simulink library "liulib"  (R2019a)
settings: Solver=ode45  StartTime=0.0  StopTime=10.0  RelTol=1e-3  EnableMultiTasking=on
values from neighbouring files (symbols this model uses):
  ag = ones(ng,1); [fPg,fTg] = bfgenD(0,P)    [bfgenD.m]    (also in fbtfit.m = AA \ [Ip ; rBt^2 ; 0]; fbtt.m = zeros(L.ng,1); fgeFpicard.m = x(2+(1:L.ng)))
  aq = []    [fbtt.m]
  aW = []    [fbtt.m]
  D = Fyi1j + Fyim1j + A.*Fyij1  +B.*Fyijm1 - C.*Fyij    [dlst.m]    (also in fbtp.m = meqp(); fgep.m = fgsp(P,varargin{:}))
  dr2FA = dr2Fs(1:nA,1)    [asxycs.m]
  drzFA = drzFs(1:nA,1)    [asxycs.m]
  dz = (z - zx(kz))/dzx    [bintc.m]
  dz2FA = dz2Fs(1:nA,1)    [asxycs.m]
  FA = Fs(1:nA,1)    [asxycs.m]    (also in bfhelp.m = [-1                        0      	 0])
  FB = [0                         1        1]    [bfhelp.m]
  Fx = zeros(n+2,3); Fx(2:end-1,2) = FN    [bfhelp.m]    (also in fbtt.m = meqFx(L,Iy,[Ia;Iu]); fgeFpicard.m = FxP + Fxe)
  FX = Fs(nA+1:ns,1)    [asxycs.m]
  Ie = [Ia;Iu]    [fgeF.m]    (also in fgeFpicard.m = (L.Mee + diag(LXt.dt*L.Re))\       ([LXt.dt*LXt.Va;zeros(L.G)
  IpD = LX.IpD(:,kt)    [fbtt.m]    (also in fgeFpicard.m = LXt.(L.agconc{1,3}))
  Iy = (Iy+flipud(Iy))*0.5    [fbtt.m]    (also in fgeF.m = reshape( xnl(L.ind.iy) , L.nzy, L.nry); fgeFpicard.m = Iyscal*reshape(Tyg*ag,L.nzy,L.nry))
  L = fbtc(P,G)    [fbt.m]    (also in fbtc.m = meqc(P,G,'rrx','zzx'); fbte.m = varargout{1}; fge.m = fgel(L,meqxk(LX,1)); fgec.m = fgsc(P,G))
  lB = false    [fbtt.m]
  lX = false    [fbtt.m]
  nA = numel(rA)    [asxycs.m]    (also in fbtt.m; fgeFpicard.m)
  niter = L.P.itercs    [asxycs.m]    (also in fbtt.m = 2)
  Opy = zeros(meqsize(L, 'Opy'),'int8')    [fbtt.m]
  rA = rs(1:nA,1)    [asxycs.m]    (also in fbtptcv.m = (rA1 + 3*rA2)/4)
  rBt = LX.rBt(kt)    [fbtt.m]    (also in fgeFpicard.m = LXt.rBt)
  rX = rs(nA+1:ns,1)    [asxycs.m]    (also in fbtptcv.m = rzbro(iX,1); fbtxana.m = r0 + [1; 1]*a0*0.5)
  zA = zs(1:nA,1)    [asxycs.m]    (also in fbtptcv.m = (zA1 + 3*zA2)/4)
  zX = zs(nA+1:ns,1)    [asxycs.m]    (also in fbtptcv.m = rzbro(iX,2); fbtxana.m = z0 + [1;-1]*a0*1.0)
undefined symbols (not defined in the file or in its folder): aminor, Bm, bp, bpli2, Brn, Brrn, Brzn, bt, Bzn, Bzrn, Bzzn, delta, deltal, deltau, dzg, epsilon, err, Ff, Fn, Ft, Ft0, FW, Ip, iqQ, iTQ, jtorQ, kappa, li, lp, mu, nX, PpQ, PQ, Q0Q, Q1Q, Q2Q, Q3Q, Q4Q, q95, qmin, raQ, raqmin, rB, rbary, repmat, rgeom, rIp, rIpD, Row, rq, rS, rst, TQ, TTpQ, vector, Vn, Vp, Wk, WN, Wp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
libraries: $bdroot x52, mkllib x48, simulink x7
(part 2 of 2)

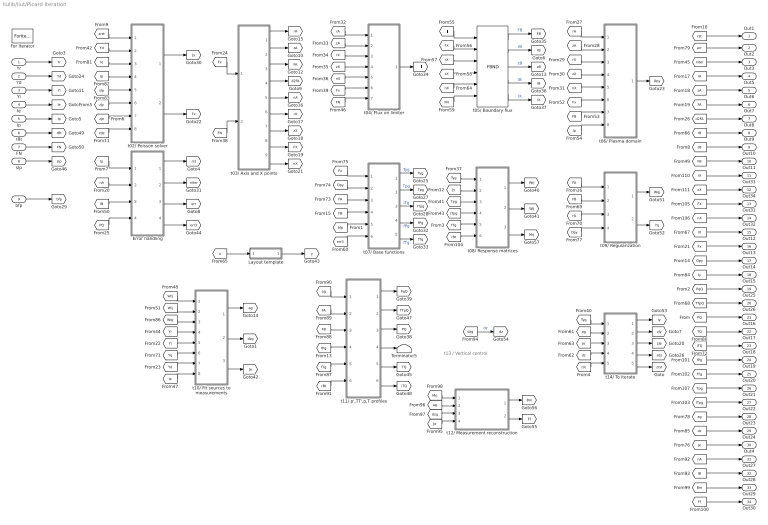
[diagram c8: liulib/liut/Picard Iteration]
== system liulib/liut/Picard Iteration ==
  note: t13 / Vertical control
  Yr : Inport
  Yd : Inport  Port=2
  Yi : Inport  Port=3
  Ie : Inport  Port=4
  Ip : Inport  Port=5
  rBt : Inport  Port=6
  FN : Inport  Port=7
  sIp : Inport  Port=8
  bfp : Inport  Port=9
  Error handling : Subsystem
  For Iterator : ForIterator  IterationLimit=L.P.itert  ShowIterationPort=off
  Layout template : Subsystem  Commented=on
  Terminator5 : Terminator
  t02/ Poisson solver : Subsystem
  t03/ Axis and X points : Subsystem  TreatAsAtomicUnit=on
  t04/ Flux on limiter : Subsystem
  t05/ Boundary flux : $bdroot/FBND  rl=L.G.rl  zl=L.G.zl
  t06/ Plasma domain : Subsystem
  t07/ Base functions : Subsystem  Variant=on
  t08/ Response matrices : Subsystem
  t09/ Regularization : Subsystem  TreatAsAtomicUnit=on
  t10/ Fit sources to measurements : Subsystem  Variant=on  VariantControl=Variant1
  t11/ p',TT',p,T profiles : Subsystem  VariantControl=Variant1
  t12/ Measurement reconstruction : Subsystem
  t14/ To iterate : Subsystem
  Out1 : Outport
  Out2 : Outport  Port=2
  Out3 : Outport  Port=3
  Out5 : Outport  Port=4
  Out6 : Outport  Port=5
  Out7 : Outport  Port=6
  Out8 : Outport  Port=7
  Out9 : Outport  Port=8
  Out10 : Outport  Port=9
  Out11 : Outport  Port=10
  Out33 : Outport  Port=11
  Out34 : Outport  Port=12
  Out31 : Outport  Port=13
  Out32 : Outport  Port=14
  Out12 : Outport  Port=15
  Out13 : Outport  Port=16
  Out14 : Outport  Port=17
  Out15 : Outport  Port=18
  Out25 : Outport  Port=19
  Out26 : Outport  Port=20
  Out16 : Outport  Port=21
  Out17 : Outport  Port=22
  Out18 : Outport  Port=23
  Out19 : Outport  Port=24
  Out20 : Outport  Port=25
  Out21 : Outport  Port=26
  Out22 : Outport  Port=27
  Out23 : Outport  Port=28
  Out24 : Outport  Port=29
  Out4 : Outport  Port=30
  Out27 : Outport  Port=31
  Out28 : Outport  Port=32
  Out29 : Outport  Port=33
  Out30 : Outport  Port=34
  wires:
  t03/ Axis and X points/9(nX) -> [nX]
  t03/ Axis and X points/8(FX) -> [FX]
  t03/ Axis and X points/7(zX) -> [zX]
  t03/ Axis and X points/6(rX) -> [rX]
  t03/ Axis and X points/5(nA) -> [nA]
  t03/ Axis and X points/4(d2FA) -> [d2FA]
  t03/ Axis and X points/3(FA) -> [FA]
  t03/ Axis and X points/2(zA) -> [zA]
  t03/ Axis and X points/1(rA) -> [rA]
  [FN] -> t03/ Axis and X points/2(FN)
  [Fx] -> t03/ Axis and X points/1(Fx)
  [zX] -> Out34/1
  [rX] -> Out33/1
  [nX] -> Out32/1
  [Bm] -> Out29/1
  [Ff] -> Out30/1
  [Je] -> t12/ Measurement reconstruction/4(Ie)
  t08/ Response matrices/3(Mrj) -> [Mrj]
  [dzg] -> t12/ Measurement reconstruction/3(dzg)
  [ag] -> t12/ Measurement reconstruction/2(ag)
  [Mrj] -> t12/ Measurement reconstruction/1(Mrj)
  t12/ Measurement reconstruction/2(Ff) -> [Ff]
  t12/ Measurement reconstruction/1(Bm) -> [Bm]
  [dzg] -> [dz]  "dz"
  [lB] -> Out28/1
  [nA] -> Out27/1
  t14/ To iterate/1(Iy) -> [Iy]
  [TTpQ] -> Out26/1
  [PqQ] -> Out25/1
  t14/ To iterate/5(zrst) -> [zrst]
  t14/ To iterate/4(zdz) -> [zdz]
  t14/ To iterate/3(zJe) -> [zJe]
  t14/ To iterate/2(zJy) -> [zJy]
  [dz] -> t14/ To iterate/4(dz)
  [Je] -> t14/ To iterate/3(Je)
  [Tyg] -> t14/ To iterate/1(Tyg)
  [ag] -> t14/ To iterate/2(ag)
  [rst] -> t14/ To iterate/5(rst)
  [fPg] -> t11/ p',TT',p,T profiles/4(fPg)
  [ag] -> t11/ p',TT',p,T profiles/1(ag)
  [FA] -> t11/ p',TT',p,T profiles/2(FA)
  [ITpg] -> Out22/1
  rBt/1 -> [rBt]
  FN/1 -> [FN]
  [zB] -> Out10/1
  Error handling/2(niter) -> [niter]
  Error handling/1(rst) -> [rst]
  t08/ Response matrices/1(Wrj) -> [Wrj]
  [Fx] -> t07/ Base functions/1(Fx)
  [Opy] -> t07/ Base functions/2(Opy)
  [FA] -> t07/ Base functions/3(FA)
  t02/ Poisson solver/1(Jy) -> [Jy]
  [zdz] -> t02/ Poisson solver/8(zdz)
  t02/ Poisson solver/2(Fx) -> [Fx]
  [dz] -> Out24/1
  [niter] -> Out3/1
  [lB] -> Error handling/3(lB)
  Error handling/3(err) -> [err]
  [Fx] -> t06/ Plasma domain/6(Fx)
  [FB] -> t06/ Plasma domain/7(FB)
  [Ip] -> t06/ Plasma domain/8(Ip)
  [TQ] -> Out17/1
  [Ie] -> t02/ Poisson solver/3(Ie)
  [Ip] -> t02/ Poisson solver/4(Ip)
  [rBt] -> t11/ p',TT',p,T profiles/6(rBt)
  [err] -> Out2/1
  [ag] -> Out23/1
  [d2FA] -> Out8/1
  [FA] -> Out7/1
  [FB] -> t07/ Base functions/4(FB)
  [err3] -> t07/ Base functions/6(err)
  t07/ Base functions/1(Tyg) -> [Tyg]  "Tyg"
  [bfp] -> t07/ Base functions/5(bfp)
  t07/ Base functions/4(fPg) -> [fPg]  "fPg"
  t07/ Base functions/5(fTg) -> [fTg]  "fTg"
  t05/ Boundary flux/1 -> [FB]  "FB"
  t05/ Boundary flux/2 -> [rB]  "rB"
  t05/ Boundary flux/3 -> [zB]  "zB"
  t05/ Boundary flux/4 -> [lB]  "lB"
  sIp/1 -> [sIp]
  [sIp] -> t02/ Poisson solver/5(sIp)
  [rst] -> Out1/1
  [Jy] -> t08/ Response matrices/2(Jy)
  t06/ Plasma domain/1(Opy) -> [Opy]
  [Tyg] -> t08/ Response matrices/1(Tyg)
  [Tpg] -> t08/ Response matrices/3(Tpg)
  t11/ p',TT',p,T profiles/1(PpQ) -> [PqQ]
  t11/ p',TT',p,T profiles/2(TTpQ) -> [TTpQ]
  t11/ p',TT',p,T profiles/4(hqTQ) -> Terminator5/1
  [fTg] -> t08/ Response matrices/5(fTg)
  t08/ Response matrices/2(Wij) -> [Wij]
  [zA] -> t06/ Plasma domain/2(zA)
  [zX] -> t06/ Plasma domain/4(zX)
  [nX] -> t06/ Plasma domain/5(nX)
  t11/ p',TT',p,T profiles/5(TQ) -> [TQ]
  t11/ p',TT',p,T profiles/6(iTQ) -> [iTQ]
  [iTQ] -> Out18/1
  [zJy] -> t02/ Poisson solver/6(zJy)
  [Yd] -> t02/ Poisson solver/2(Yd)
  [zJe] -> t02/ Poisson solver/7(zJe)
  Yr/1 -> [Yr]
  Yi/1 -> [Yi]
  Ip/1 -> [Ip]
  bfp/1 -> [bfp]
  [FN] -> t04/ Flux on limiter/7(FN)
  [Fx] -> t04/ Flux on limiter/6(Fx)
  [Fl] -> t05/ Boundary flux/1
  Yd/1 -> [Yd]
  Ie/1 -> [Ie]
  [zrst] -> t02/ Poisson solver/1(rst)
  [FB] -> t11/ p',TT',p,T profiles/3(FB)
  [fTg] -> t11/ p',TT',p,T profiles/5(fTg)
  t05/ Boundary flux/5 -> [lX]  "lX"
  [rA] -> t06/ Plasma domain/1(rA)
  [rX] -> t06/ Plasma domain/3(rX)
  [zX] -> t04/ Flux on limiter/4(zX)
  [rX] -> t04/ Flux on limiter/3(rX)
  [nX] -> t04/ Flux on limiter/5(nX)
  [Tpg] -> Out21/1
  [fTg] -> Out20/1
  [fPg] -> Out19/1
  [ITpg] -> t08/ Response matrices/4(ITpg)
  t04/ Flux on limiter/1(Fl) -> [Fl]
  [zA] -> Out6/1
  [rA] -> Out5/1
  [nX] -> t05/ Boundary flux/5
  [rB] -> Out9/1
  [lX] -> Out12/1
  t11/ p',TT',p,T profiles/3(PQ) -> [PQ]
  [Opy] -> Out14/1
  [FB] -> Out11/1
  [Fx] -> Out13/1
  [Ip] -> Error handling/1(Ip)
  [nA] -> Error handling/2(nA)
  [PQ] -> Error handling/4(PQ)
  [Iy] -> Out15/1
  [PQ] -> Out16/1
  [rX] -> t05/ Boundary flux/3
  [FX] -> t05/ Boundary flux/2
  [zX] -> t05/ Boundary flux/4
  Layout template/1(y) -> [y]
  [u] -> Layout template/1(u)
  [FN] -> t05/ Boundary flux/6
  [rA] -> t04/ Flux on limiter/1(rA)
  [zA] -> t04/ Flux on limiter/2(zA)
  t07/ Base functions/2(Tpg) -> [Tpg]  "Tpg"
  t07/ Base functions/3(ITpg) -> [ITpg]  "iTg"
  Error handling/4(err3) -> [err3]
  [Wrj] -> t10/ Fit sources to measurements/1(Wrj)
  [Wij] -> t10/ Fit sources to measurements/2(Wij)
  [Yr] -> t10/ Fit sources to measurements/4(Yr)
  [Yi] -> t10/ Fit sources to measurements/5(Yi)
  [Yd] -> t10/ Fit sources to measurements/7(Yd)
  [Ie] -> t10/ Fit sources to measurements/8(Ie)
  t10/ Fit sources to measurements/1(ag) -> [ag]
  t10/ Fit sources to measurements/2(dzg) -> [dzg]
  t10/ Fit sources to measurements/3(Je) -> [Je]
  t09/ Regularization/1(Wqj) -> [Wqj]
  t09/ Regularization/2(Yq) -> [Yq]
  [rA] -> t09/ Regularization/3(rA)
  [Opy] -> t09/ Regularization/4(Opy)
  [FB] -> t09/ Regularization/2(FB)
  [FA] -> t09/ Regularization/1(FA)
  [Yq] -> t10/ Fit sources to measurements/6(Yq)
  [Wqj] -> t10/ Fit sources to measurements/3(Wqj)
  [Je] -> Out4/1
  [rBt] -> t08/ Response matrices/6(rBt)
  [FX] -> Out31/1

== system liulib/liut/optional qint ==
  "LY " : Inport
  Fx : Inport  Port=2
  direct pass : Subsystem  VariantControl=liuINFCTMODEvariant1
  "qint " : Subsystem  VariantControl=liuINFCTMODEvariant2
  " LYo" : Outport

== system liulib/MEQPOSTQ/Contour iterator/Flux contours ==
  zaq : Inport
  rst : Inport  Port=2
  rA : Inport  Port=3
  zA : Inport  Port=4
  FA : Inport  Port=5
  FB : Inport  Port=6
  Fx : Inport  Port=7
  Opy : Inport  Port=8
  IC=1 : UnitDelay  InitialCondition=1  SampleTime=-1  HasFrameUpgradeWarning=on
  Opo : Constant  Value=int8(1)
  RTCI : $bdroot/RTCI  c=L.cdrq  s=L.cdzq  da=L.drx  nr=L.nrx  nz=L.nzx
  Sum : Sum  Inputs=|+-
  Sum1 : Sum  Inputs=|+-
  Sum5 : Sum  Inputs=|+-
  "aq " : Switch  Criteria=u2 ~= 0
  aq0 : Subsystem  TreatAsAtomicUnit=on
  dan : Terminator
  fq : Gain  Gain=L.fq  ParamDataTypeStr=single  OutDataTypeStr=single
  idrx : Gain  Gain=L.idrx  ParamDataTypeStr=single  OutDataTypeStr=single
  idzx : Gain  Gain=L.idzx  ParamDataTypeStr=single  OutDataTypeStr=single
  qaq3 : Sum  Inputs=|++
  rx1 : Constant  Value=L.G.rx(1)  OutDataTypeStr=single
  zx1 : Constant  Value=L.G.zx(1)  OutDataTypeStr=single
  aq : Outport
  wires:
  qaq3/1 -> RTCI/5
  Fx/1 -> RTCI/4
  idzx/1 -> RTCI/3
  idrx/1 -> RTCI/2
  RTCI/2 -> dan/1
  zaq/1 -> "aq "/3
  aq0/1(aq) -> "aq "/1
  "aq "/1 -> RTCI/1
  rA/1 -> Sum/1, aq0/1(rA)
  rx1/1 -> Sum/2
  Sum/1 -> idrx/1
  zA/1 -> Sum1/1, aq0/2(zA)
  zx1/1 -> Sum1/2
  Sum1/1 -> idzx/1
  Sum5/1 -> fq/1
  fq/1 -> qaq3/1
  FB/1 -> Sum5/2, qaq3/2
  FA/1 -> RTCI/7, Sum5/1
  RTCI/1 -> aq/1  "aq"
  Opy/1 -> RTCI/6
  Opo/1 -> RTCI/8
  rst/1 -> IC=1/1
  IC=1/1 -> aq0/Enable, "aq "/2

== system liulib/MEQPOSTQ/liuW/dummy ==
  LY : Inport
  LYo : Outport
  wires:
  LY/1 -> LYo/1

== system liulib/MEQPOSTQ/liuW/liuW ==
  LY : Inport
  Bus Assignment : BusAssignment  AssignedSignals=aW,FW
  Bus Selector : BusSelector  OutputSignals=rst,Fx,Opy,FB,FX,lX,nX
  MATLAB Function : MATLAB Function  TreatAsAtomicUnit=on  mask{nFW=L.P.nFW}
  liuW : Subsystem  VariantControl=liuAWMODEvariant1
  LYo : Outport
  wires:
  Bus Selector/7 -> MATLAB Function/4(nX)  "<nX>"
  Bus Selector/6 -> MATLAB Function/3(lX)  "<lX>"
  Bus Selector/5 -> MATLAB Function/2(FX)  "<FX>"
  Bus Selector/4 -> MATLAB Function/1(FB)  "<FB>"
  Bus Selector/2 -> liuW/2(Fx)  "<Fx>"
  Bus Selector/3 -> liuW/3(Opy)  "<Opy>"
  Bus Selector/1 -> liuW/1(rst)  "<rst>"
  LY/1 -> Bus Selector/1, Bus Assignment/1
  MATLAB Function/1(FW) -> Bus Assignment/3, liuW/4(FW)
  liuW/1(aW) -> Bus Assignment/2
  Bus Assignment/1 -> LYo/1

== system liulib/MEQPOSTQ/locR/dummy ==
  LY : Inport
  "raQ " : Inport  Port=2
  "qQ " : Inport  Port=3
  sq : Inport  Port=4
  Terminator : Terminator
  Terminator1 : Terminator
  Terminator2 : Terminator
  " LYo" : Outport
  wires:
  "raQ "/1 -> Terminator/1
  "qQ "/1 -> Terminator1/1
  sq/1 -> Terminator2/1
  LY/1 -> " LYo"/1

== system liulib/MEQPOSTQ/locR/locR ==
  LY : Inport
  raQ : Inport  Port=2
  qQ : Inport  Port=3
  sq : Inport  Port=4
  Apply sign : Product  Inputs=**
  Bus Assignment : BusAssignment  AssignedSignals=raR
  Constant3 : Constant  Value=L.P.iqR  OutDataTypeStr=single
  Constant4 : Constant  Value=L.raN  OutDataTypeStr=single
  locR : $bdroot/locR  nR=L.nR  naR=L.P.naR
  " LYo" : Outport
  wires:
  Constant4/1 -> locR/4
  qQ/1 -> locR/2
  sq/1 -> Apply sign/2
  Apply sign/1 -> locR/3
  raQ/1 -> locR/1
  Constant3/1 -> Apply sign/1
  locR/1 -> Bus Assignment/2  "raR"
  LY/1 -> Bus Assignment/1
  Bus Assignment/1 -> " LYo"/1

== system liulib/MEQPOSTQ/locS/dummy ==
  "LY " : Inport
  " LYo" : Outport
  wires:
  "LY "/1 -> " LYo"/1

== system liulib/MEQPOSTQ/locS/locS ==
  LY : Inport
  Bus Assignment4 : BusAssignment  AssignedSignals=rS,zS
  Bus Selector : BusSelector  OutputSignals=aq,raQ,rA,zA
  Constant1 : Constant  Value=L.P.raS  OutDataTypeStr=single
  Constant2 : Constant  Value=L.raN  OutDataTypeStr=single
  Matrix Concatenate : Concatenate  Mode=Multidimensional array  ConcatenateDimension=2
  RTCI1 : $bdroot/RTCI1  SFunctionModules=''
  RTCI2 : $bdroot/RTCI1  SFunctionModules=''
  crq : Constant  Value=L.crq  OutDataTypeStr=single
  czq : Constant  Value=L.czq  OutDataTypeStr=single
  locS : $bdroot/locS  SFunctionModules=''
  row of zeros : Constant  Value=zeros(L.noq,1)  OutDataTypeStr=Inherit: Inherit via back propagation
  LYo : Outport
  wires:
  Bus Selector/4 -> RTCI2/3  "<zA>"
  Bus Assignment4/1 -> LYo/1
  LY/1 -> Bus Selector/1, Bus Assignment4/1
  locS/1 -> RTCI1/1, RTCI2/1
  Matrix Concatenate/1 -> locS/1
  Bus Selector/2 -> locS/2  "<raQ>"
  Constant1/1 -> locS/3
  czq/1 -> RTCI2/2
  crq/1 -> RTCI1/2
  Bus Selector/3 -> RTCI1/3  "<rA>"
  RTCI2/1 -> Bus Assignment4/3
  RTCI1/1 -> Bus Assignment4/2
  Constant2/1 -> locS/4
  row of zeros/1 -> Matrix Concatenate/1
  Bus Selector/1 -> Matrix Concatenate/2  "<aq>"

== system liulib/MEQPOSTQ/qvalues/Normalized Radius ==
  aq : Inport
  Constant : Constant  Value=0  OutDataTypeStr=single
  Normalise : Product  Inputs=*/
  Outboard radius : Selector  NumberOfDimensions=2  InputPortWidth=3  IndexOptions=Index vector (dialog),Select all  Indices=find(L.crq==1),L.npq  OutputSizes=1,1
  Permute Dimensions : PermuteDimensions
  Reshape : Reshape
  Reshape1 : Reshape
  Vector Concatenate : Concatenate
  end value : Selector  InputPortWidth=L.npq  IndexOptions=Index vector (dialog)  Indices=L.npq  OutputSizes=1
  raQ : Outport
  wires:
  Outboard radius/1 -> Reshape1/1
  Reshape1/1 -> end value/1, Normalise/1
  Constant/1 -> Vector Concatenate/1
  aq/1 -> Outboard radius/1
  Normalise/1 -> Vector Concatenate/2
  end value/1 -> Normalise/2
  Reshape/1 -> raQ/1
  Permute Dimensions/1 -> Reshape/1
  Vector Concatenate/1 -> Permute Dimensions/1

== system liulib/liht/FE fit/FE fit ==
  Yd : Inport
  Ie : Inport  Port=2
  Ip_in : Inport  Port=3
  sIp : Inport  Port=4
  FE : $bdroot/FE  SystemSampleTime=-1
  Iph : mkllib/A*u  A=L.Iph
  Iph_D : mkllib/A*u  A=[L.Iph_t;L.Iph_b]
  Iprh : mkllib/A*u  A=L.Iprh
  Iprh_D : mkllib/A*u  A=[L.Iprh_t;L.Iprh_b]
  Ipzh : mkllib/A*u  A=L.Ipzh
  Ipzh_D : mkllib/A*u  A=[L.Ipzh_t;L.Ipzh_b]
  Subsystem1 : Subsystem
  Variant Source : VariantSource
  Variant Source1 : VariantSource
  Variant Source2 : VariantSource
  Je : Outport
  IpD : Outport  Port=2
  rIpD : Outport  Port=3
  zIpD : Outport  Port=4
  Ip : Outport  Port=5
  rIp : Outport  Port=6
  zIp : Outport  Port=7
  rA : Outport  Port=8
  zA : Outport  Port=9
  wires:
  Variant Source2/1 -> zIpD/1, Subsystem1/3(zIp)
  Variant Source1/1 -> Subsystem1/2(rIp), rIpD/1  "rIpD"
  Variant Source/1 -> IpD/1, Subsystem1/1(Ip)
  Subsystem1/1(rA) -> rA/1  "rA"
  Subsystem1/2(zA) -> zA/1  "zA"
  FE/2 -> Je/1
  sIp/1 -> FE/4
  Yd/1 -> FE/1
  Ip_in/1 -> FE/3
  Ie/1 -> FE/2
  Iprh_D/1 -> Variant Source1/1  "rIpD"
  FE/1 -> Iph_D/1, Ipzh/1, Iprh/1, Iph/1, Ipzh_D/1, Iprh_D/1
  Iph_D/1 -> Variant Source/1  "IpD"
  Ipzh_D/1 -> Variant Source2/1  "zIpD"
  Iprh/1 -> rIp/1, Variant Source1/2  "rIp"
  Iph/1 -> Ip/1, Variant Source/2  "Ip"
  Ipzh/1 -> zIp/1, Variant Source2/2  "zIp"

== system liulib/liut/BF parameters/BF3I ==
  BF3I parameters : Subsystem
  Bus Creator : BusCreator  Inputs=4
  bfp : Outport
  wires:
  BF3I parameters/2(IgNg) -> Bus Creator/2
  BF3I parameters/4(fTg) -> Bus Creator/4
  BF3I parameters/3(fPg) -> Bus Creator/3
  Bus Creator/1 -> bfp/1
  BF3I parameters/1(gNg) -> Bus Creator/1

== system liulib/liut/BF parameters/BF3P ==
  Constant : Constant  Value=L.P.bfp
  bfp : Outport
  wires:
  Constant/1 -> bfp/1

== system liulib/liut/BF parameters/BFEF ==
  Constant : Constant  Value=L.P.bfp
  bfp : Outport
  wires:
  Constant/1 -> bfp/1

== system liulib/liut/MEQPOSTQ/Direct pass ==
  "LY " : Inport
  "sIp " : Inport  Port=2
  Terminator : Terminator
  " LYo" : Outport
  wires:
  "LY "/1 -> " LYo"/1
  "sIp "/1 -> Terminator/1

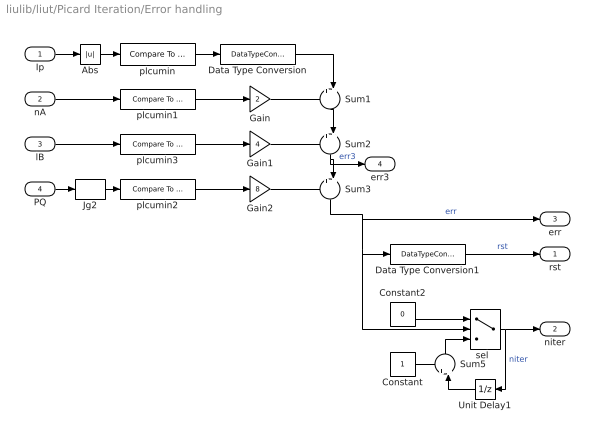
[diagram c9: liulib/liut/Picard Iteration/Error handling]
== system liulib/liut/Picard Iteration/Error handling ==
  Ip : Inport
  nA : Inport  Port=2
  lB : Inport  Port=3
  PQ : Inport  Port=4
  Abs : Abs
  Constant : Constant  VectorParams1D=off  OutDataTypeStr=int32
  Constant2 : Constant  Value=0  VectorParams1D=off  OutDataTypeStr=int32
  Data Type Conversion : DataTypeConversion  OutDataTypeStr=int32
  Data Type Conversion1 : DataTypeConversion  OutDataTypeStr=boolean
  Gain : Gain  Gain=2  OutDataTypeStr=int32
  Gain1 : Gain  Gain=4  OutDataTypeStr=int32
  Gain2 : Gain  Gain=8  OutDataTypeStr=int32
  Jg2 : Selector  IndexMode=Zero-based  IndexOptions=Index vector (dialog)  Indices=0  OutputSizes=1
  Sum{1..3,5} (4 alike) : Sum  Inputs=++|
  Unit Delay1 : UnitDelay  InitialCondition=int32(0)  SampleTime=-1  HasFrameUpgradeWarning=on
  plcumin : simulink/Logic and Bit Operations/Compare To Constant  relop=<  const=L.P.Ipmin  OutDataTypeStr=uint8
  plcumin1 : simulink/Logic and Bit Operations/Compare To Constant  relop===  const=0  OutDataTypeStr=uint8
  plcumin2 : simulink/Logic and Bit Operations/Compare To Constant  relop=<  const=0  OutDataTypeStr=uint8
  plcumin3 : simulink/Logic and Bit Operations/Compare To Constant  relop===  const=0  OutDataTypeStr=uint8
  "sel  " : Switch  Criteria=u2 ~= 0  OutDataTypeStr=int32
  rst : Outport
  niter : Outport  Port=2
  err : Outport  Port=3
  err3 : Outport  Port=4
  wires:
  plcumin2/1 -> Gain2/1
  nA/1 -> plcumin1/1
  Jg2/1 -> plcumin2/1
  PQ/1 -> Jg2/1
  Data Type Conversion1/1 -> rst/1  "rst"
  Ip/1 -> Abs/1
  Abs/1 -> plcumin/1
  "sel  "/1 -> niter/1, Unit Delay1/1  "niter"
  Sum5/1 -> "sel  "/3
  Constant/1 -> Sum5/1
  lB/1 -> plcumin3/1
  plcumin3/1 -> Gain1/1
  Unit Delay1/1 -> Sum5/2
  Constant2/1 -> "sel  "/1
  plcumin1/1 -> Gain/1
  plcumin/1 -> Data Type Conversion/1
  Gain1/1 -> Sum2/1
  Gain2/1 -> Sum3/1
  Sum3/1 -> "sel  "/2, Data Type Conversion1/1, err/1  "err"
  Gain/1 -> Sum1/1
  Data Type Conversion/1 -> Sum1/2
  Sum1/1 -> Sum2/2
  Sum2/1 -> err3/1, Sum3/2  "err3"

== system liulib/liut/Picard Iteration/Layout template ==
  u : Inport
  y : Outport
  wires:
  u/1 -> y/1

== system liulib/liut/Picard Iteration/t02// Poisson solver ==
  rst : Inport
  Yd : Inport  Port=2
  Ie : Inport  Port=3
  Ip : Inport  Port=4
  sIp : Inport  Port=5
  zJy : Inport  Port=6
  zJe : Inport  Port=7
  zdz : Inport  Port=8
  *idzx : Gain  Gain=single(L.idzx)
  Constant2 : Constant  Value=0  OutDataTypeStr=single
  Fb : Switch  Criteria=u2 ~= 0
  Fb BF : Subsystem  TreatAsAtomicUnit=on
  Fb FE : Subsystem  TreatAsAtomicUnit=on
  GSZR : $bdroot/GSZR  cx=L.cx  cq=L.cq  cr=L.cr  cs=L.cs  ci=L.ci  co=L.co  bc=1
  Je : Switch  Criteria=u2 ~= 0
  Jw : $bdroot/ASGN  iu=L.kyw-1
  "Jy " : Switch  Criteria=u2 ~= 0
  KYWMODE : VariantSource
  Logical Operator : Logic  Operator=NOT  IconShape=distinctive  AllPortsSameDT=off  OutDataTypeStr=boolean
  Mbe : mkllib/A*u  A=L.Mbe
  Sum3 : Sum
  Tww : mkllib/A*u  A=single(L.Tww)
  dz : Switch  Criteria=u2 ~= 0
  kew : Selector  IndexMode=Zero-based  IndexOptions=Index vector (dialog)  Indices=L.kew-1  OutputSizes=1
  Jy : Outport
  Fx : Outport  Port=2
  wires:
  Yd/1 -> Fb FE/1(Yd)
  GSZR/1 -> Fx/1  "Fx"
  zdz/1 -> dz/3, Fb BF/3(dz)  "zdz"
  zJe/1 -> Fb BF/2(Je)  "zJe"
  kew/1 -> Tww/1
  rst/1 -> Fb FE/Enable, Fb/2, Je/2, dz/2, Logical Operator/1, "Jy "/2
  Logical Operator/1 -> Fb BF/Enable
  zJy/1 -> Fb BF/1(Jy)  "zJy"
  Mbe/1 -> Sum3/2
  Je/1 -> Mbe/1, kew/1
  Fb/1 -> Sum3/1  "Fb"
  "Jy "/1 -> Jw/1, KYWMODE/1, Jy/1  "Jy"
  Fb FE/3(Je) -> Je/1
  Fb FE/2(Fb) -> Fb/1
  Fb BF/2(Fb) -> Fb/3
  Tww/1 -> Jw/2
  Fb FE/1(Jy) -> "Jy "/1
  dz/1 -> *idzx/1
  Constant2/1 -> dz/1
  Ie/1 -> Fb FE/2(Ie)
  Ip/1 -> Fb FE/3(Ip)
  sIp/1 -> Fb FE/4(sIp)
  Fb BF/3(=Je) -> Je/3
  Fb BF/1(=Jy) -> "Jy "/3
  Jw/1 -> KYWMODE/2
  KYWMODE/1 -> GSZR/1
  Sum3/1 -> GSZR/2
  *idzx/1 -> GSZR/3

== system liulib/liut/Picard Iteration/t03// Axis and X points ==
  Fx : Inport
  FN : Inport  Port=2
  ASXY : $bdroot/ASXY  rx=L.G.rx  zx=L.G.zx  dr=L.drx  dz=L.dzx  idr=L.idrx  idz=L.idzx  Oasx=L.Oasx  daxm=L.P.dasm
  Terminator{,1..3} (4 alike) : Terminator
  Vector Concatenate : Concatenate  NumInputs=3
  rA : Outport
  zA : Outport  Port=2
  FA : Outport  Port=3
  d2FA : Outport  Port=4
  nA : Outport  Port=5
  rX : Outport  Port=6
  zX : Outport  Port=7
  FX : Outport  Port=8
  nX : Outport  Port=9
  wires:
  ASXY/8 -> rX/1  "rX"
  ASXY/5 -> Vector Concatenate/2
  ASXY/10 -> FX/1  "FX"
  ASXY/9 -> zX/1  "zX"
  ASXY/4 -> Vector Concatenate/1
  Fx/1 -> ASXY/1
  ASXY/1 -> rA/1  "rA"
  ASXY/6 -> Vector Concatenate/3
  ASXY/15 -> Terminator3/1  "stat"
  ASXY/11 -> Terminator/1  "dr2FX"
  ASXY/3 -> FA/1  "FA"
  ASXY/13 -> Terminator2/1  "drzFX"
  FN/1 -> ASXY/2
  ASXY/14 -> nX/1  "nX"
  ASXY/2 -> zA/1  "zA"
  ASXY/12 -> Terminator1/1  "dz2FX"
  ASXY/7 -> nA/1  "nA"
  Vector Concatenate/1 -> d2FA/1  "d2FA"

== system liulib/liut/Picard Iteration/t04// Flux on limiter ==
  rA : Inport
  zA : Inport  Port=2
  rX : Inport  Port=3
  zX : Inport  Port=4
  nX : Inport  Port=5
  Fx : Inport  Port=6
  FN : Inport  Port=7
  Constant : Constant  Value=L.G.rl  OutDataTypeStr=single
  Constant1 : Constant  Value=L.G.zl  OutDataTypeStr=single
  FL4P1 : $bdroot/FL4P  kl=int32(L.kxl-1)  cl=L.clx  nz=L.nzx
  Sum : Sum  Inputs=-+|
  Sum1 : Sum  Inputs=-+|
  Switch : Switch  Criteria=u2 ~= 0
  l in OX : $bdroot/l in OX1  a=0
  Fl : Outport
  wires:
  Switch/1 -> Fl/1
  nX/1 -> l in OX/5
  l in OX/1 -> Switch/2
  FL4P1/1 -> Switch/1
  rX/1 -> Sum/1, l in OX/1
  zX/1 -> Sum1/1, l in OX/2
  rA/1 -> FL4P1/5, Sum/2
  Sum/1 -> l in OX/3
  zA/1 -> FL4P1/6, Sum1/2
  Sum1/1 -> l in OX/4
  Fx/1 -> FL4P1/1
  FN/1 -> Switch/3, FL4P1/2
  Constant/1 -> l in OX/6, FL4P1/3
  Constant1/1 -> FL4P1/4, l in OX/7

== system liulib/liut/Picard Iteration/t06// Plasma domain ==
  rA : Inport
  zA : Inport  Port=2
  rX : Inport  Port=3
  zX : Inport  Port=4
  nX : Inport  Port=5
  Fx : Inport  Port=6
  FB : Inport  Port=7
  Ip : Inport  Port=8
  Constant : Constant  Value=L.ry  OutDataTypeStr=Inherit: Inherit via back propagation
  Constant1 : Constant  Value=L.zy  OutDataTypeStr=Inherit: Inherit via back propagation
  Data Type Conversion : DataTypeConversion  OutDataTypeStr=int8
  OXy : $bdroot/BAVX2  a=0
  PDOM : $bdroot/PDOM
  Sum : Sum  Inputs=-+|
  Sum1 : Sum  Inputs=-+|
  Opy : Outport
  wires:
  Fx/1 -> PDOM/1
  FB/1 -> PDOM/2
  Ip/1 -> PDOM/3
  nX/1 -> OXy/5
  OXy/1 -> PDOM/4
  Constant1/1 -> OXy/7
  Constant/1 -> OXy/6
  rX/1 -> Sum/1, OXy/1
  zX/1 -> Sum1/1, OXy/2
  rA/1 -> Sum/2
  Sum/1 -> OXy/3
  Sum1/1 -> OXy/4
  zA/1 -> Sum1/2
  PDOM/1 -> Data Type Conversion/1  "Opy"
  Data Type Conversion/1 -> Opy/1

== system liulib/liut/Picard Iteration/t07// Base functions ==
  Fx : Inport
  Opy : Inport  Port=2
  FA : Inport  Port=3
  FB : Inport  Port=4
  bfp : Inport  Port=5
  err : Inport  Port=6
  bf3i : Subsystem  VariantControl=liuBFCTMODEvariant2
  bf3p : Subsystem  VariantControl=liuBFCTMODEvariant1
  bfef : Subsystem  VariantControl=liuBFCTMODEvariant3
  Tyg : Outport
  Tpg : Outport  Port=2
  ITpg : Outport  Port=3
  fPg : Outport  Port=4
  fTg : Outport  Port=5

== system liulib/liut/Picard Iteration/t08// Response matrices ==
  Tyg : Inport
  Jy : Inport  Port=2
  Tpg : Inport  Port=3
  ITpg : Inport  Port=4
  fTg : Inport  Port=5
  rBt : Inport  Port=6
  Add : Sum
  Constant1 : Constant  Value=L.Mty  OutDataTypeStr=single
  Gain : Gain  Gain=repmat(L.Wr,1,L.nj)
  Product : Product  Inputs=3
  Product1 : Product
  Reshape : Reshape  OutputDimensionality=Row vector (2-D)
  Wi j : Concatenate  Mode=Multidimensional array  ConcatenateDimension=2
  Wp : Gain  Gain=L.Wp
  Wriz : Concatenate  Mode=Multidimensional array
  Wt : Gain  Gain=L.Wt
  "[0;0]" : Constant  Value=[0;0]  OutDataTypeStr=single
  "[Mry*Tyg Mdzry*Jy]" : $bdroot/RESP  A=L.Mry  B=L.Mdzry  nr=L.nr  ng=L.ng
  mu0/2pi : Constant  Value=single(2e-7)  OutDataTypeStr=single
  v*U : mkllib/v*U  alpha=1  order=102  transA=112  incx=1  beta=0  incy=1
  Wrj : Outport
  Wij : Outport  Port=2
  Mrj : Outport  Port=3
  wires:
  Gain/1 -> Wrj/1
  ITpg/1 -> Product/1
  Tpg/1 -> Wp/1
  Wp/1 -> Wriz/2
  Wt/1 -> Wriz/1
  Wriz/1 -> Wi j/1
  "[0;0]"/1 -> Wi j/2
  Wi j/1 -> Wij/1
  "[Mry*Tyg Mdzry*Jy]"/1 -> Gain/1, Mrj/1
  fTg/1 -> Product/2
  Jy/1 -> "[Mry*Tyg Mdzry*Jy]"/2
  Tyg/1 -> v*U/1, "[Mry*Tyg Mdzry*Jy]"/1
  mu0/2pi/1 -> Product/3
  v*U/1 -> Product1/1
  rBt/1 -> Product1/2
  Product1/1 -> Reshape/1
  Add/1 -> Wt/1
  Product/1 -> Add/2
  Constant1/1 -> v*U/2
  Reshape/1 -> Add/1

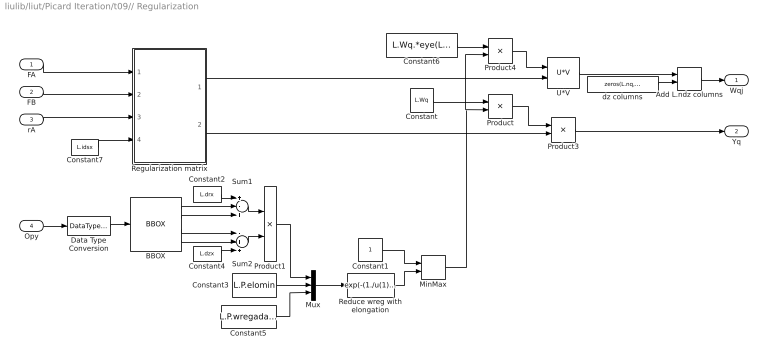
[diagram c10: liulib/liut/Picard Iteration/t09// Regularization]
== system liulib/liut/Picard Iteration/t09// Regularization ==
  FA : Inport
  FB : Inport  Port=2
  rA : Inport  Port=3
  Opy : Inport  Port=4
  Add L.ndz columns : Concatenate  Mode=Multidimensional array  ConcatenateDimension=2
  BBOX : $bdroot/BBOX  z=L.zy  r=L.ry
  Constant : Constant  Value=L.Wq  OutDataTypeStr=single
  Constant1 : Constant  OutDataTypeStr=single
  Constant2 : Constant  Value=L.drx  OutDataTypeStr=single
  Constant3 : Constant  Value=L.P.elomin  OutDataTypeStr=single
  Constant4 : Constant  Value=L.dzx  OutDataTypeStr=single
  Constant5 : Constant  Value=L.P.wregadapt  OutDataTypeStr=single
  Constant6 : Constant  Value=L.Wq.*eye(L.nq)  OutDataTypeStr=single
  Constant7 : Constant  Value=L.idsx  OutDataTypeStr=single
  Data Type Conversion : DataTypeConversion  OutDataTypeStr=boolean
  MinMax : MinMax  Inputs=2
  Mux : Mux  Inputs=3
  Product : Product
  Product1 : Product  Inputs=*/
  Product3 : Product
  Product4 : Product
  Reduce wreg with elongation : Fcn  Expr=exp(-(1./u(1)-u(2))*u(3))
  Regularization matrix : Subsystem  Variant=on  VariantControl=Variant1
  Sum1 : Sum  Inputs=+-+
  Sum2 : Sum  Inputs=-++
  U*V : mkllib/U*V  a=1
  dz columns : Constant  Value=zeros(L.nq,L.ndz)  OutDataTypeStr=single
  Wqj : Outport
  Yq : Outport  Port=2
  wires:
  FA/1 -> Regularization matrix/1("FA ")
  FB/1 -> Regularization matrix/2("FB ")
  rA/1 -> Regularization matrix/3("rA ")
  Constant7/1 -> Regularization matrix/4("ids ")
  BBOX/1 -> Sum1/2
  Sum2/1 -> Product1/2
  Constant2/1 -> Sum1/1
  Sum1/1 -> Product1/1
  BBOX/4 -> Sum2/2
  BBOX/2 -> Sum1/3
  Constant4/1 -> Sum2/3
  BBOX/3 -> Sum2/1
  Reduce wreg with elongation/1 -> MinMax/2
  Constant/1 -> Product/1
  Product3/1 -> Yq/1
  U*V/1 -> Add L.ndz columns/1
  Add L.ndz columns/1 -> Wqj/1
  Constant1/1 -> MinMax/1
  MinMax/1 -> Product4/2, Product/2
  Mux/1 -> Reduce wreg with elongation/1
  Constant6/1 -> Product4/1
  Product/1 -> Product3/1
  Regularization matrix/2(" Xq") -> Product3/2
  Product4/1 -> U*V/1
  Regularization matrix/1(" Qqg") -> U*V/2
  Product1/1 -> Mux/1
  Constant3/1 -> Mux/2
  Constant5/1 -> Mux/3
  Opy/1 -> Data Type Conversion/1
  Data Type Conversion/1 -> BBOX/1
  dz columns/1 -> Add L.ndz columns/2

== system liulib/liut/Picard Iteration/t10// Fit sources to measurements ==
  Wrj : Inport
  Wij : Inport  Port=2
  Wqj : Inport  Port=3
  Yr : Inport  Port=4
  Yi : Inport  Port=5
  Yq : Inport  Port=6
  Yd : Inport  Port=7
  Ie : Inport  Port=8
  Double precision : Subsystem  VariantControl=liuBSLVMODEvariant2
  Single precision : Subsystem  VariantControl=liuBSLVMODEvariant1
  ag : Outport
  dzg : Outport  Port=2
  Je : Outport  Port=3

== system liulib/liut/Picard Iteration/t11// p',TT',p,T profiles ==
  ag : Inport
  FA : Inport  Port=2
  FB : Inport  Port=3
  fPg : Inport  Port=4
  fTg : Inport  Port=5
  rBt : Inport  Port=6
  Small diamagnetism approximation : Subsystem
  p',TT',p,hqT profiles : Subsystem  VariantControl=BFCTMODE==1
  PpQ : Outport
  TTpQ : Outport  Port=2
  PQ : Outport  Port=3
  hqTQ : Outport  Port=4
  TQ : Outport  Port=5
  iTQ : Outport  Port=6
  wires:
  fPg/1 -> p',TT',p,hqT profiles/4(fPg)
  ag/1 -> p',TT',p,hqT profiles/1(ag)
  Small diamagnetism approximation/2(iT) -> iTQ/1  "iTQ"
  Small diamagnetism approximation/1(T) -> TQ/1  "TQ"
  rBt/1 -> Small diamagnetism approximation/2(rBt)
  p',TT',p,hqT profiles/4(hqTQ) -> Small diamagnetism approximation/1(hqT), hqTQ/1
  FA/1 -> p',TT',p,hqT profiles/2(FA)
  p',TT',p,hqT profiles/1(PpQ) -> PpQ/1
  p',TT',p,hqT profiles/2(TTpQ) -> TTpQ/1
  p',TT',p,hqT profiles/3(PQ) -> PQ/1
  FB/1 -> p',TT',p,hqT profiles/3(FB)
  fTg/1 -> p',TT',p,hqT profiles/5(fTg)

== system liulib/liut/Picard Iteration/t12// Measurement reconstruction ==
  Mrj : Inport
  ag : Inport  Port=2
  dzg : Inport  Port=3
  Ie : Inport  Port=4
  1/fdz : Gain  Gain=1/L.P.fdz
  Add : Sum
  Gain : Gain  Gain=L.Mre  Multiplication=Matrix(K*u) (u vector)
  Selector : Selector  IndexOptions=Index vector (dialog)  Indices=1:L.G.nf  OutputSizes=1
  Selector1 : Selector  IndexOptions=Index vector (dialog)  Indices=L.G.nf + (1:L.G.nm)  OutputSizes=1
  U*v : mkllib/U*v  a=1
  Vector Concatenate : Concatenate
  Bm : Outport
  Ff : Outport  Port=2
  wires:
  Selector/1 -> Ff/1  "Ff"
  Selector1/1 -> Bm/1  "Bm"
  Add/1 -> Selector/1, Selector1/1
  Gain/1 -> Add/2
  Ie/1 -> Gain/1
  U*v/1 -> Add/1
  Mrj/1 -> U*v/1
  Vector Concatenate/1 -> U*v/2  "aj"
  dzg/1 -> 1/fdz/1
  ag/1 -> Vector Concatenate/1
  1/fdz/1 -> Vector Concatenate/2

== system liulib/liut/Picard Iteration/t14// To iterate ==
  Tyg : Inport
  ag : Inport  Port=2
  Je : Inport  Port=3
  dz : Inport  Port=4
  rst : Inport  Port=5
  Jx : mkllib/U*v  a=1
  Unit Delay : UnitDelay  InitialCondition=1  SampleTime=-1  HasFrameUpgradeWarning=on
  Unit Delay1 : UnitDelay  SampleTime=-1  HasFrameUpgradeWarning=on
  Unit Delay2 : UnitDelay  SampleTime=-1  HasFrameUpgradeWarning=on
  Unit Delay4 : UnitDelay  SampleTime=-1  HasFrameUpgradeWarning=on
  Iy : Outport
  zJy : Outport  Port=2
  zJe : Outport  Port=3
  zdz : Outport  Port=4
  zrst : Outport  Port=5
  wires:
  rst/1 -> Unit Delay/1
  Unit Delay/1 -> zrst/1
  Je/1 -> Unit Delay2/1
  Unit Delay2/1 -> zJe/1
  ag/1 -> Jx/2
  dz/1 -> Unit Delay1/1
  Tyg/1 -> Jx/1
  Jx/1 -> Unit Delay4/1, Iy/1  "Iy"
  Unit Delay4/1 -> zJy/1
  Unit Delay1/1 -> zdz/1

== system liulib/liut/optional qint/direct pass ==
  LY : Inport
  Fx : Inport  Port=2
  Terminator : Terminator
  LYo : Outport
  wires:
  Fx/1 -> Terminator/1
  LY/1 -> LYo/1

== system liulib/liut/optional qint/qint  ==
  note: Loop voltage calculation at interpolation points by Finite Differences
  LY : Inport
  Fx : Inport  Port=2
  Add : Sum  Inputs=+-
  Bus Assignment3 : BusAssignment  AssignedSignals=Fn,Brn,Bzn,Brrn,Brzn,Bzrn,Bzzn,Vn
  Constant1 : Constant  Value=single(L.P.rn)
  Constant2 : Constant  Value=single(L.P.zn)
  Gain : Gain  Gain=single(1/L.dt)
  Memory : Memory
  QINT : $bdroot/QINT  rx=L.rx  zx=L.zx  inM=L.inM
  Switch : Switch  Criteria=u2 ~= 0
  LYo : Outport
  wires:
  Gain/1 -> Switch/1
  Switch/1 -> Bus Assignment3/9
  Add/1 -> Gain/1
  QINT/1 -> Bus Assignment3/2, Add/1, Memory/1
  Memory/1 -> Add/2, Switch/2, Switch/3
  Fx/1 -> QINT/1
  QINT/7 -> Bus Assignment3/8
  QINT/6 -> Bus Assignment3/7
  QINT/5 -> Bus Assignment3/6
  QINT/4 -> Bus Assignment3/5
  QINT/3 -> Bus Assignment3/4
  QINT/2 -> Bus Assignment3/3
  Constant2/1 -> QINT/3
  Constant1/1 -> QINT/2
  LY/1 -> Bus Assignment3/1
  Bus Assignment3/1 -> LYo/1

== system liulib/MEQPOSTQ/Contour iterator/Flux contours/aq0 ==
  rA : Inport
  zA : Inport  Port=2
  rst : EnablePort
  Sum{,1..3} (4 alike) : Sum  Inputs=|+-
  a1 : MinMax  Inputs=4
  pq0 : Gain  Gain=L.pinit*repmat(L.pq,L.noq,1)
  rx1 : Constant  Value=L.G.rx(1)  OutDataTypeStr=single
  rx9 : Constant  Value=L.G.rx(end)  OutDataTypeStr=single
  zx1 : Constant  Value=L.G.zx(1)  OutDataTypeStr=single
  zx9 : Constant  Value=L.G.zx(end)  OutDataTypeStr=single
  aq : Outport
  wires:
  a1/1 -> pq0/1
  Sum2/1 -> a1/4
  Sum3/1 -> a1/3
  Sum/1 -> a1/2
  Sum1/1 -> a1/1
  zx9/1 -> Sum3/1
  zA/1 -> Sum2/1, Sum3/2
  zx1/1 -> Sum2/2
  rx9/1 -> Sum1/1
  rA/1 -> Sum1/2, Sum/1
  rx1/1 -> Sum/2
  pq0/1 -> aq/1

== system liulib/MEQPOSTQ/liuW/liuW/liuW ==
  rst : Inport
  Fx : Inport  Port=2
  Opy : Inport  Port=3
  FW : Inport  Port=4
  For Iterator : ForIterator  IterationLimit=L.P.iterq  ShowIterationPort=off
  Unit Delay : UnitDelay  SampleTime=-1  HasFrameUpgradeWarning=on
  liuW : $bdroot/liuW  SystemSampleTime=-1
  aW : Outport
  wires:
  Opy/1 -> liuW/5
  Fx/1 -> liuW/4
  FW/1 -> liuW/3
  rst/1 -> liuW/2
  Unit Delay/1 -> liuW/1
  liuW/1 -> aW/1, Unit Delay/1

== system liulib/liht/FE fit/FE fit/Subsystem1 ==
  Ip : Inport
  rIp : Inport  Port=2
  zIp : Inport  Port=3
  Constant : Constant  Value=0  OutDataTypeStr=Inherit: Inherit via back propagation
  Divide2 : Product  Inputs=*/
  Divide3 : Product  Inputs=*/
  Switch2 : Switch  Criteria=u2 ~= 0
  Switch3 : Switch  Criteria=u2 ~= 0
  rA : Outport
  zA : Outport  Port=2
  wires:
  Switch3/1 -> zA/1
  rIp/1 -> Divide2/1
  Divide3/1 -> Switch3/1
  Switch2/1 -> rA/1
  Constant/1 -> Switch3/3, Switch2/3
  zIp/1 -> Divide3/1
  Ip/1 -> Divide2/2, Switch2/2, Switch3/2, Divide3/2
  Divide2/1 -> Switch2/1

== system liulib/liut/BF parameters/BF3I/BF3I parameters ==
  Constant : Constant  Value=L.P.bfp.gNg  VectorParams1D=off  OutDataTypeStr=single
  Constant1 : Constant  Value=L.P.bfp.IgNg  VectorParams1D=off  OutDataTypeStr=single
  Constant2 : Constant  Value=L.P.bfp.fPg  OutDataTypeStr=single
  Constant3 : Constant  Value=L.P.bfp.fTg  OutDataTypeStr=single
  gNg : Outport
  IgNg : Outport  Port=2
  fPg : Outport  Port=3
  fTg : Outport  Port=4
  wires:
  Constant/1 -> gNg/1
  Constant3/1 -> fTg/1
  Constant2/1 -> fPg/1
  Constant1/1 -> IgNg/1

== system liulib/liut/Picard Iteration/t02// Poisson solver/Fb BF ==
  Jy : Inport
  Je : Inport  Port=2
  dz : Inport  Port=3
  ~rst : EnablePort
  Add : Sum  Inputs=+-
  Constant : Constant  Value=0  OutDataTypeStr=single
  Constant1 : Constant  Value=zeros(1,(L.nzy+L.nry)*2+4)  OutDataTypeStr=single
  Divide : Product  Inputs=**
  GSZR BC=0 : Subsystem  TreatAsAtomicUnit=on
  NFDB : $bdroot/NFDB  nz=L.nzx  nr=L.nrx
  Tbc : mkllib/A*u  A=single(L.Tbc)
  dzMbe : mkllib/A*u  A=single(L.dzMbe)
  =Jy : Outport
  Fb : Outport  Port=2
  =Je : Outport  Port=3
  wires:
  Jy/1 -> GSZR BC=0/1(Iy), =Jy/1
  dzMbe/1 -> Add/2
  Add/1 -> Fb/1
  Divide/1 -> dzMbe/1
  dz/1 -> Divide/2
  Je/1 -> =Je/1, Divide/1
  Tbc/1 -> Add/1
  NFDB/1 -> Tbc/1
  Constant1/1 -> GSZR BC=0/2(Fb)
  Constant/1 -> GSZR BC=0/3(dz)
  GSZR BC=0/1(Fx) -> NFDB/1

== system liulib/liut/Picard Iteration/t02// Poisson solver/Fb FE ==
  Yd : Inport
  Ie : Inport  Port=2
  Ip : Inport  Port=3
  sIp : Inport  Port=4
  rst : EnablePort
  FE : $bdroot/FE  SystemSampleTime=-1
  Mbh* : mkllib/A*u  A=L.Mbh
  Tyh* : mkllib/A*u  A=L.Tyh
  Jy : Outport
  Fb : Outport  Port=2
  Je : Outport  Port=3
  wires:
  Mbh*/1 -> Fb/1
  Tyh*/1 -> Jy/1
  Yd/1 -> FE/1
  FE/2 -> Je/1
  Ie/1 -> FE/2
  Ip/1 -> FE/3
  sIp/1 -> FE/4
  FE/1 -> Mbh*/1, Tyh*/1

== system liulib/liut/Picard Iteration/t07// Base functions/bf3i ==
  Fx : Inport
  Opy : Inport  Port=2
  FA : Inport  Port=3
  FB : Inport  Port=4
  bfp : Inport  Port=5
  err : Inport  Port=6
  BF3I1 : $bdroot/BF3I1  r=L.ry  ir=L.iry  nz=L.nzy  nr=L.nry
  Demux : Demux  BusSelectionMode=on
  Tyg : Outport
  Tpg : Outport  Port=2
  ITpg : Outport  Port=3
  fPg : Outport  Port=4
  fTg : Outport  Port=5
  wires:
  Fx/1 -> BF3I1/1
  Opy/1 -> BF3I1/2
  FA/1 -> BF3I1/3
  FB/1 -> BF3I1/4
  BF3I1/1 -> Tyg/1
  BF3I1/2 -> Tpg/1
  BF3I1/3 -> ITpg/1
  Demux/1 -> BF3I1/5
  Demux/2 -> BF3I1/6
  Demux/3 -> BF3I1/7, fPg/1
  bfp/1 -> Demux/1
  Demux/4 -> fTg/1, BF3I1/8
  err/1 -> BF3I1/9

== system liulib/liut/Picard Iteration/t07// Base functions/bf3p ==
  Fx : Inport
  Opy : Inport  Port=2
  FA : Inport  Port=3
  FB : Inport  Port=4
  bfp : Inport  Port=5
  err : Inport  Port=6
  BF3P1 : $bdroot/BF3P1  ry=L.ry  iry=L.iry  nzy=L.nzy  nry=L.nry
  Constant : Constant  Value=[1 0 0]  VectorParams1D=off  OutDataTypeStr=single
  Constant1 : Constant  Value=[0 1 1]  VectorParams1D=off  OutDataTypeStr=single
  Constant2 : Constant  Value=false
  Terminator : Terminator
  Tyg : Outport
  Tpg : Outport  Port=2
  ITpg : Outport  Port=3
  fPg : Outport  Port=4
  fTg : Outport  Port=5
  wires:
  err/1 -> BF3P1/6
  FB/1 -> BF3P1/4
  FA/1 -> BF3P1/3
  Fx/1 -> BF3P1/1
  BF3P1/1 -> Tyg/1
  BF3P1/3 -> ITpg/1
  BF3P1/2 -> Tpg/1
  Constant2/1 -> BF3P1/5
  Opy/1 -> BF3P1/2
  bfp/1 -> Terminator/1
  Constant/1 -> fPg/1
  Constant1/1 -> fTg/1

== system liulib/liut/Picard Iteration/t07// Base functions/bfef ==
  Fx : Inport
  Opy : Inport  Port=2
  FA : Inport  Port=3
  FB : Inport  Port=4
  bfp : Inport  Port=5
  err : Inport  Port=6
  BFEF1 : $bdroot/BFEF1  ry=L.ry  iry=L.iry  nzy=L.nzy  nry=L.nry  nP=L.P.bfp(1)  nT=L.P.bfp(2)
  Constant1 : Constant  Value=L.fTg  OutDataTypeStr=single
  Constant2 : Constant  Value=L.fPg  OutDataTypeStr=single
  Terminator : Terminator
  Tyg : Outport
  Tpg : Outport  Port=2
  ITpg : Outport  Port=3
  fPg : Outport  Port=4
  fTg : Outport  Port=5
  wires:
  Fx/1 -> BFEF1/1
  Opy/1 -> BFEF1/2
  FA/1 -> BFEF1/3
  FB/1 -> BFEF1/4
  err/1 -> BFEF1/5
  BFEF1/3 -> ITpg/1
  BFEF1/2 -> Tpg/1
  BFEF1/1 -> Tyg/1
  Constant2/1 -> fPg/1
  Constant1/1 -> fTg/1
  bfp/1 -> Terminator/1

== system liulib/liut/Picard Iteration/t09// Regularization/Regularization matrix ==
  "FA " : Inport
  "FB " : Inport  Port=2
  "rA " : Inport  Port=3
  "ids " : Inport  Port=4
  bf3i : Subsystem  VariantControl=liuBFCTMODEvariant2
  bf3p : Subsystem  VariantControl=liuBFCTMODEvariant1
  bfef : Subsystem  VariantControl=liuBFCTMODEvariant3
  " Qqg" : Outport
  " Xq" : Outport  Port=2

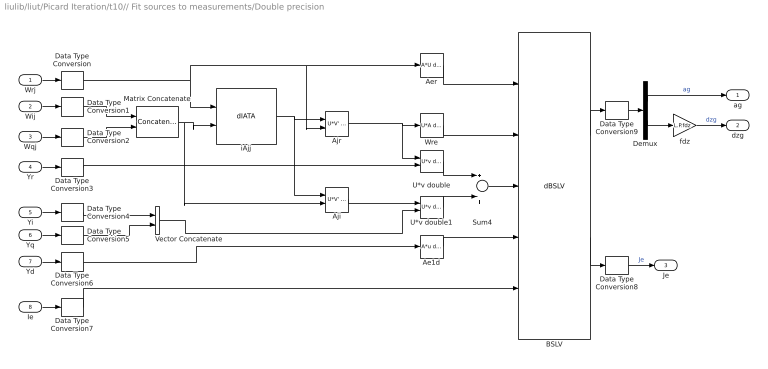
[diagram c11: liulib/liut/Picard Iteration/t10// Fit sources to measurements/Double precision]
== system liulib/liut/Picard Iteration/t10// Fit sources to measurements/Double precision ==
  Wrj : Inport
  Wij : Inport  Port=2
  Wqj : Inport  Port=3
  Yr : Inport  Port=4
  Yi : Inport  Port=5
  Yq : Inport  Port=6
  Yd : Inport  Port=7
  Ie : Inport  Port=8
  Ae1d : mkllib/A*u double  A=L.Ae1d
  Aer : mkllib/A*U double  A=L.Aer
  Aji : mkllib/U*V' double  a=1
  Ajr : mkllib/U*V' double  a=1
  BSLV : $bdroot/dBSLV  niter=L.P.iters
  Data Type Conversion{,1..7} (8 alike) : DataTypeConversion  OutDataTypeStr=double
  Data Type Conversion8 : DataTypeConversion  OutDataTypeStr=single
  Data Type Conversion9 : DataTypeConversion  OutDataTypeStr=single
  Demux : Demux  Outputs=[L.ng L.ndz]
  Matrix Concatenate : Concatenate  Mode=Multidimensional array
  Sum4 : Sum  Inputs=+|+
  U*v double : mkllib/U*v double  a=1
  U*v double1 : mkllib/U*v double  a=1
  Vector Concatenate : Concatenate
  Wre : mkllib/U*A double  A=L.Wre
  fdz : Gain  Gain=L.P.fdz
  iAjj : $bdroot/dIATA  SFunctionModules=''
  ag : Outport
  dzg : Outport  Port=2
  Je : Outport  Port=3
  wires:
  Wij/1 -> Data Type Conversion1/1
  Wrj/1 -> Data Type Conversion/1
  Yd/1 -> Data Type Conversion6/1
  Yi/1 -> Data Type Conversion4/1
  Ajr/1 -> U*v double/1, Wre/1
  BSLV/2 -> Data Type Conversion8/1
  Ae1d/1 -> BSLV/4
  Wre/1 -> BSLV/2
  Aer/1 -> BSLV/1
  Ie/1 -> Data Type Conversion7/1
  Demux/2 -> fdz/1
  Demux/1 -> ag/1  "ag"
  BSLV/1 -> Data Type Conversion9/1
  Yr/1 -> Data Type Conversion3/1
  Aji/1 -> U*v double1/1
  U*v double/1 -> Sum4/1
  U*v double1/1 -> Sum4/2
  Sum4/1 -> BSLV/3
  iAjj/1 -> Ajr/1, Aji/1
  fdz/1 -> dzg/1  "dzg"
  Data Type Conversion/1 -> iAjj/1, Ajr/2, Aer/1
  Data Type Conversion3/1 -> U*v double/2
  Data Type Conversion6/1 -> Ae1d/1
  Data Type Conversion7/1 -> BSLV/5
  Data Type Conversion8/1 -> Je/1  "Je"
  Data Type Conversion9/1 -> Demux/1
  Yq/1 -> Data Type Conversion5/1
  Wqj/1 -> Data Type Conversion2/1
  Data Type Conversion1/1 -> Matrix Concatenate/1
  Data Type Conversion2/1 -> Matrix Concatenate/2
  Matrix Concatenate/1 -> Aji/2, iAjj/2
  Data Type Conversion4/1 -> Vector Concatenate/1
  Data Type Conversion5/1 -> Vector Concatenate/2
  Vector Concatenate/1 -> U*v double1/2

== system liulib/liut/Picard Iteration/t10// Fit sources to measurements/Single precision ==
  Wrj : Inport
  Wij : Inport  Port=2
  Wqj : Inport  Port=3
  Yr : Inport  Port=4
  Yi : Inport  Port=5
  Yq : Inport  Port=6
  Yd : Inport  Port=7
  Ie : Inport  Port=8
  Ae1d : mkllib/A*u  A=L.Ae1d
  Aer : mkllib/A*U  A=L.Aer
  Aji : mkllib/U*V'  a=1
  Ajr : mkllib/U*V'  a=1
  BSLV : $bdroot/sBSLV  niter=L.P.iters
  Demux : Demux  Outputs=[L.ng L.ndz]
  Matrix Concatenate : Concatenate  Mode=Multidimensional array
  Sum4 : Sum  Inputs=+|+
  Vector Concatenate : Concatenate
  Wre : mkllib/U*A  A=L.Wre
  fdz : Gain  Gain=L.P.fdz
  iAjj : $bdroot/sIATA  SFunctionModules=''
  xg1 : mkllib/U*v  a=1
  xg2 : mkllib/U*v  a=1
  ag : Outport
  dzg : Outport  Port=2
  Je : Outport  Port=3
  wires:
  Wrj/1 -> iAjj/1, Aer/1, Ajr/2
  Yd/1 -> Ae1d/1
  Ajr/1 -> xg1/1, Wre/1
  BSLV/2 -> Je/1  "Je"
  Ae1d/1 -> BSLV/4
  Wre/1 -> BSLV/2
  Aer/1 -> BSLV/1
  Ie/1 -> BSLV/5
  Demux/2 -> fdz/1
  Demux/1 -> ag/1  "ag"
  BSLV/1 -> Demux/1
  Yr/1 -> xg1/2
  Aji/1 -> xg2/1
  xg1/1 -> Sum4/1
  xg2/1 -> Sum4/2
  Sum4/1 -> BSLV/3
  iAjj/1 -> Aji/1, Ajr/1
  fdz/1 -> dzg/1  "dz"
  Matrix Concatenate/1 -> Aji/2, iAjj/2
  Wij/1 -> Matrix Concatenate/1
  Wqj/1 -> Matrix Concatenate/2
  Yi/1 -> Vector Concatenate/1
  Yq/1 -> Vector Concatenate/2
  Vector Concatenate/1 -> xg2/2

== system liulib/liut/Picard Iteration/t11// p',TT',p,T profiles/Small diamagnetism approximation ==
  hqT : Inport
  rBt : Inport  Port=2
  Constant : Constant  OutDataTypeStr=single
  Constant1 : Constant  Value=2  OutDataTypeStr=single
  Sum1 : Sum
  Sum2 : Sum  Inputs=-+
  ahqTg1 : Product
  ahqTg2 : Product
  ahqTg3 : Product
  irBt : Product  Inputs=/*
  T : Outport
  iT : Outport  Port=2
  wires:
  ahqTg2/1 -> Sum2/1
  Constant1/1 -> Sum2/2
  irBt/1 -> ahqTg2/2, ahqTg3/2, ahqTg1/2
  Sum1/1 -> ahqTg2/1, T/1
  Constant/1 -> irBt/2
  ahqTg1/1 -> Sum1/1
  rBt/1 -> irBt/1, Sum1/2
  hqT/1 -> ahqTg1/1
  ahqTg3/1 -> iT/1
  Sum2/1 -> ahqTg3/1

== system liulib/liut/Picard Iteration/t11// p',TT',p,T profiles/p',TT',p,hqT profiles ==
  ag : Inport
  FA : Inport  Port=2
  FB : Inport  Port=3
  fPg : Inport  Port=4
  fTg : Inport  Port=5
  Base functions on rho grid Coefficients for source terms : Subsystem  Variant=on
  Constant : Constant  Value=L.TQg  VectorParams1D=off  OutDataTypeStr=single
  Constant1 : Constant  Value=L.ITQg  VectorParams1D=off  OutDataTypeStr=single
  smvunv{,1..3} (4 alike) : mkllib/U*v  a=1
  PpQ : Outport
  TTpQ : Outport  Port=2
  PQ : Outport  Port=3
  hqTQ : Outport  Port=4
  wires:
  smvunv2/1 -> PQ/1  "PQ"
  smvunv/1 -> PpQ/1  "PpQ"
  Constant1/1 -> smvunv3/1, smvunv2/1
  FA/1 -> Base functions on rho grid Coefficients for source terms/2(FA)
  FB/1 -> Base functions on rho grid Coefficients for source terms/3(FB)
  ag/1 -> Base functions on rho grid Coefficients for source terms/1(ag)
  Base functions on rho grid Coefficients for source terms/1(aPpg) -> smvunv/2
  Base functions on rho grid Coefficients for source terms/2(aTTpg) -> smvunv1/2
  Base functions on rho grid Coefficients for source terms/3(aPg) -> smvunv2/2
  Base functions on rho grid Coefficients for source terms/4(ahqTg) -> smvunv3/2
  fPg/1 -> Base functions on rho grid Coefficients for source terms/4(fPg)
  fTg/1 -> Base functions on rho grid Coefficients for source terms/5(fTg)
  smvunv3/1 -> hqTQ/1  "hqTQ"
  smvunv1/1 -> TTpQ/1  "TTpQ"
  Constant/1 -> smvunv1/1, smvunv/1

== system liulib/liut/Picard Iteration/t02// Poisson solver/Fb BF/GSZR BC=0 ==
  note: This subsystem is mecessary to allow treating this as an atomic subsystem. Otherwise we would get improper real-time behaviour
  Iy : Inport
  Fb : Inport  Port=2
  dz : Inport  Port=3
  GSZR : $bdroot/GSZR  cx=L.cx  cq=L.cq  cr=L.cr  cs=L.cs  ci=L.ci  co=L.co  bc=0
  Fx : Outport
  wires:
  dz/1 -> GSZR/3
  Iy/1 -> GSZR/1
  Fb/1 -> GSZR/2
  GSZR/1 -> Fx/1

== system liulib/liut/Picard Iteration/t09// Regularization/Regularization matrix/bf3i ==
  "FA " : Inport
  "FB " : Inport  Port=2
  "rA " : Inport  Port=3
  "ids " : Inport  Port=4
  BF3I6 : $bdroot/BF3I6  SFunctionModules=''
  Terminator{,1..3} (4 alike) : Terminator
  " Qqg" : Outport
  " Xq" : Outport  Port=2
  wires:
  BF3I6/1 -> " Qqg"/1
  BF3I6/2 -> " Xq"/1
  "FA "/1 -> Terminator/1
  "FB "/1 -> Terminator1/1
  "rA "/1 -> Terminator2/1
  "ids "/1 -> Terminator3/1

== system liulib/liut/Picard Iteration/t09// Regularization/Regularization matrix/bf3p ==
  "FA " : Inport
  "FB " : Inport  Port=2
  "rA " : Inport  Port=3
  "ids " : Inport  Port=4
  BF3P6 : $bdroot/BF3P6  SFunctionModules=''
  Divide : Product  Inputs=/
  " Qqg" : Outport
  " Xq" : Outport  Port=2
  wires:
  "FA "/1 -> BF3P6/1
  "FB "/1 -> BF3P6/2
  Divide/1 -> BF3P6/3
  "ids "/1 -> BF3P6/4
  BF3P6/2 -> " Xq"/1
  BF3P6/1 -> " Qqg"/1
  "rA "/1 -> Divide/1

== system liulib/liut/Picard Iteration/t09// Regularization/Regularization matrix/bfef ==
  "FA " : Inport
  "FB " : Inport  Port=2
  "rA " : Inport  Port=3
  "ids " : Inport  Port=4
  BFEF6 : $bdroot/BFEF6  nP=L.P.bfp(1)  nT=L.P.bfp(2)  nq=L.nq
  Divide : Product  Inputs=/
  " Qqg" : Outport
  " Xq" : Outport  Port=2
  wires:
  BFEF6/1 -> " Qqg"/1
  BFEF6/2 -> " Xq"/1
  "FA "/1 -> BFEF6/1
  "FB "/1 -> BFEF6/2
  "rA "/1 -> Divide/1, BFEF6/3
  Divide/1 -> BFEF6/4
  "ids "/1 -> BFEF6/5

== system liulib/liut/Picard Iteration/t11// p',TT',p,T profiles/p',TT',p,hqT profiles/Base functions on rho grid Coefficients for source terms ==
  ag : Inport
  FA : Inport  Port=2
  FB : Inport  Port=3
  fPg : Inport  Port=4
  fTg : Inport  Port=5
  bf3i : Subsystem  VariantControl=liuBFCTMODEvariant2
  bf3p : Subsystem  VariantControl=liuBFCTMODEvariant1
  bfef : Subsystem  VariantControl=liuBFCTMODEvariant3
  aPpg : Outport
  aTTpg : Outport  Port=2
  aPg : Outport  Port=3
  ahqTg : Outport  Port=4

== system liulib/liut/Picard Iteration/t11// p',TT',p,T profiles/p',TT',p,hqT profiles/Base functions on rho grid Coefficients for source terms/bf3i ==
  ag : Inport
  FA : Inport  Port=2
  FB : Inport  Port=3
  fPg : Inport  Port=4
  fTg : Inport  Port=5
  BF3I3 : $bdroot/BF3I3  idsx=L.idsx
  aPpg : Outport
  aTTpg : Outport  Port=2
  aPg : Outport  Port=3
  ahqTg : Outport  Port=4
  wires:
  fPg/1 -> BF3I3/4
  fTg/1 -> BF3I3/5
  ag/1 -> BF3I3/1
  FA/1 -> BF3I3/2
  FB/1 -> BF3I3/3
  BF3I3/1 -> aPpg/1
  BF3I3/2 -> aTTpg/1
  BF3I3/3 -> aPg/1
  BF3I3/4 -> ahqTg/1

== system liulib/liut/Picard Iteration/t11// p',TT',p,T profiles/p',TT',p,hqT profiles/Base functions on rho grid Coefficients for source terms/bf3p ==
  ag : Inport
  FA : Inport  Port=2
  FB : Inport  Port=3
  fPg : Inport  Port=4
  fTg : Inport  Port=5
  BF3P3 : $bdroot/BF3P3  idsx=L.idsx
  Terminator1 : Terminator
  Terminator2 : Terminator
  aPpg : Outport
  aTTpg : Outport  Port=2
  aPg : Outport  Port=3
  ahqTg : Outport  Port=4
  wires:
  BF3P3/4 -> ahqTg/1
  BF3P3/3 -> aPg/1
  BF3P3/2 -> aTTpg/1
  BF3P3/1 -> aPpg/1
  FB/1 -> BF3P3/3
  FA/1 -> BF3P3/2
  ag/1 -> BF3P3/1
  fTg/1 -> Terminator1/1
  fPg/1 -> Terminator2/1

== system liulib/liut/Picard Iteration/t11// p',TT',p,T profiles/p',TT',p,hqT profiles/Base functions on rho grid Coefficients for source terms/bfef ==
  ag : Inport
  FA : Inport  Port=2
  FB : Inport  Port=3
  fPg : Inport  Port=4
  fTg : Inport  Port=5
  BFEF3 : $bdroot/BFEF3  ids=L.idsx  nP=L.P.bfp(1)  nT=L.P.bfp(2)
  Terminator : Terminator
  Terminator1 : Terminator
  aPpg : Outport
  aTTpg : Outport  Port=2
  aPg : Outport  Port=3
  ahqTg : Outport  Port=4
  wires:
  ag/1 -> BFEF3/1
  FA/1 -> BFEF3/2
  FB/1 -> BFEF3/3
  BFEF3/1 -> aPpg/1
  BFEF3/2 -> aTTpg/1
  BFEF3/3 -> aPg/1
  BFEF3/4 -> ahqTg/1
  fPg/1 -> Terminator/1
  fTg/1 -> Terminator1/1

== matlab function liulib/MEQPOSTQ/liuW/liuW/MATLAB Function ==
function FW = meqFW(FB,FX,lX,nX,nFW)

FW = meqFW(FB,FX(1:nX),lX,nX,nFW);

end
